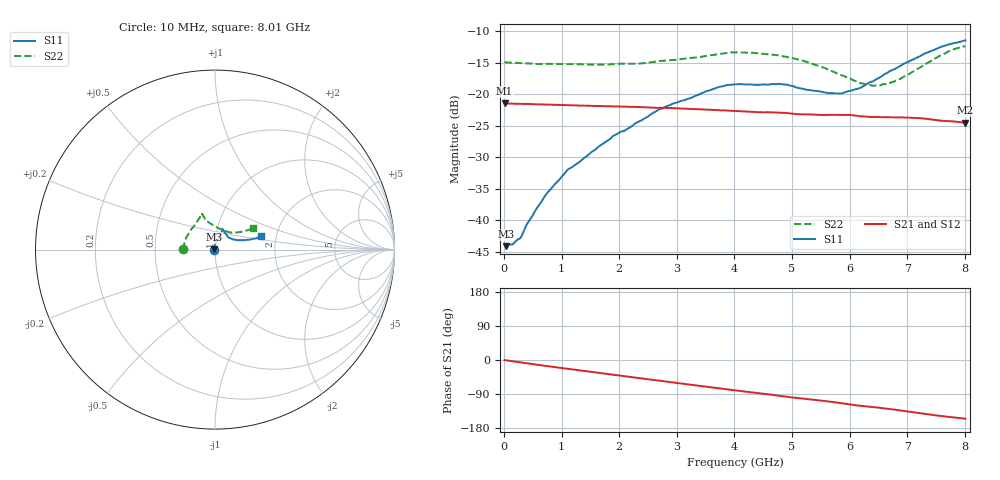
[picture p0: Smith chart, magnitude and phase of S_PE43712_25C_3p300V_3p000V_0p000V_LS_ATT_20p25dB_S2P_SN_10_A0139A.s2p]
! DEVICE ID: PE43712
! File Path: z:\PE43713\PE43713_CHAR_NOM_04292014\AMB\3p300\LS_ATT_20p25dB\PE43713_AMB_3p300V_3p000V_0p000V_LS_ATT_20p25dB_S2P_SN_10_A0139A.s2p
! Serial: 10
! Lot: A0139A
! Temp: 25C
! VDD: 3.300
! VSS: 0.000
! Control_Hi: 3.000
! Control_Lo: 0.000
! Attenuation Step: 20.25dB
! Port 1: RF1
! Port 2: RF2
! ThroughPath:1-2
! IDD: 0.0001468957
! ISS: -1.071e-007
#  Hz  S  RI  R  50
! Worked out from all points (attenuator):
!   801 points, 10 MHz to 8.01 GHz, reference 50 ohm
!   highest |S21| = -21.48 dB at 10 MHz (marker M1); lowest = -24.5 dB at 8.01 GHz (marker M2)
!   lowest |S11| = -44.1 dB at 30 MHz (marker M3), VSWR 1.01, Z = 49.4 + j0.136 ohm
!   |S11| at or under -10 dB: start of sweep to end of sweep
!   |S22| runs from -18.7 to -12.4 dB; largest |S21 - S12| = 0.00031
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1e7  -0.00647 0.000557  0.0843 -0.000392  0.0844 -0.000397  -0.1793 0.00115
3e7  -0.00608 0.00138  0.0843 -0.00106  0.0843 -0.00106  -0.1787 0.00289
1.5e8  -0.00527 0.00374  0.0839 -0.00496  0.084 -0.00498  -0.1771 0.0108
2.7e8  -0.00456 0.0055  0.0834 -0.00875  0.0834 -0.00879  -0.1755 0.0171
4.2e8  -0.00422 0.00871  0.0826 -0.0134  0.0825 -0.0134  -0.1734 0.0251
7.4e8  -0.00389 0.0158  0.0796 -0.0226  0.0796 -0.0227  -0.1683 0.0439
1.1e9  -0.00248 0.0249  0.0751 -0.0321  0.0751 -0.0321  -0.161 0.0636
1.35e9  -2.72e-05 0.0301  0.0717 -0.0382  0.0716 -0.0382  -0.1551 0.0753
1.91e9  0.00867 0.0463  0.0621 -0.0504  0.0621 -0.0504  -0.1369 0.1066
2.68e9  0.0267 0.0705  0.0457 -0.0631  0.0457 -0.0631  -0.1061 0.1494
3.71e9  0.0388 0.1063  0.0202 -0.0719  0.0201 -0.0719  -0.0814 0.1905
4.01e9  0.04 0.1127  0.0128 -0.0725  0.0128 -0.0725  -0.0807 0.1991
4.79e9  0.0437 0.1125  -0.00563 -0.0711  -0.00561 -0.0711  -0.0678 0.1904
5.35e9  0.0562 0.091  -0.0173 -0.0667  -0.0173 -0.0667  -0.0526 0.1666
5.87e9  0.0769 0.0667  -0.0279 -0.0625  -0.0278 -0.0625  -0.0165 0.1398
6.17e9  0.0952 0.058  -0.034 -0.0577  -0.0339 -0.0577  0.0122 0.1226
6.38e9  0.1123 0.0556  -0.0367 -0.0548  -0.0366 -0.0548  0.0358 0.1115
6.68e9  0.1412 0.0521  -0.0413 -0.0508  -0.0412 -0.0508  0.0717 0.0986
7e9  0.1706 0.0537  -0.0466 -0.0456  -0.0465 -0.0455  0.1055 0.0943
7.55e9  0.2252 0.0626  -0.052 -0.0336  -0.0519 -0.0336  0.1697 0.1051
7.81e9  0.2443 0.0702  -0.0534 -0.029  -0.0534 -0.029  0.1963 0.1142
8.01e9  0.2555 0.0764  -0.0537 -0.0252  -0.0535 -0.0254  0.2091 0.1181
